FUNCTION FC 7 : VOID
TITLE =COMANDI PROFIBUS AZIONAMENTO 7 ASPO
VERSION : 0.1

BEGIN
NETWORK
TITLE =TRASFERISCO I SEGNALI DI COMANDO
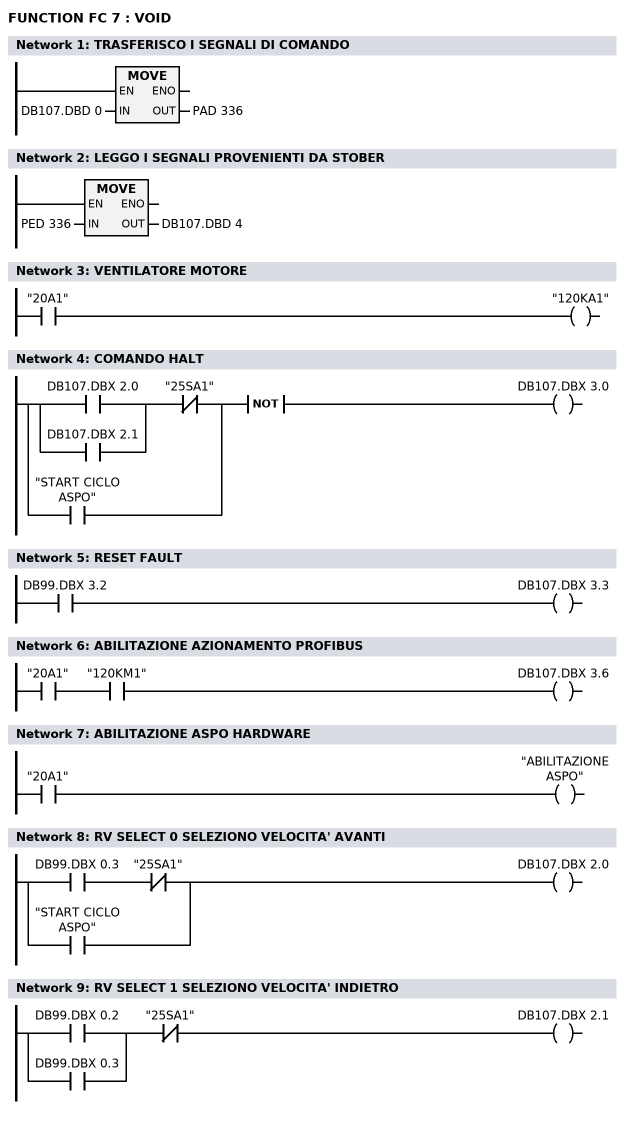
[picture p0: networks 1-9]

      L     DB107.DBD    0;
      T     PAD  336;
      NOP   0;
NETWORK
TITLE =LEGGO I SEGNALI PROVENIENTI DA STOBER

      L     PED  336;
      T     DB107.DBD    4;
      NOP   0;
NETWORK
TITLE =VENTILATORE MOTORE

      U     "20A1";
      =     "120KA1";
NETWORK
TITLE =COMANDO HALT

      U     DB107.DBX    2.0;
      O     DB107.DBX    2.1;
      UN    "25SA1";
      O     "START CICLO ASPO";
      NOT   ;
      =     DB107.DBX    3.0;
NETWORK
TITLE =RESET FAULT

      U     DB99.DBX    3.2;
      =     DB107.DBX    3.3;
NETWORK
TITLE =ABILITAZIONE AZIONAMENTO PROFIBUS

      U     "20A1";
      U     "120KM1";
      =     DB107.DBX    3.6;
NETWORK
TITLE =ABILITAZIONE ASPO HARDWARE

      U     "20A1";
      =     "ABILITAZIONE ASPO";
NETWORK
TITLE =RV SELECT 0 SELEZIONO VELOCITA' AVANTI

      U     DB99.DBX    0.3;
      UN    "25SA1";
      O     "START CICLO ASPO";
      =     DB107.DBX    2.0;
NETWORK
TITLE =RV SELECT 1 SELEZIONO VELOCITA' INDIETRO

      U     DB99.DBX    0.2;
      O     DB99.DBX    0.3;
      UN    "25SA1";
      =     DB107.DBX    2.1;
END_FUNCTION

